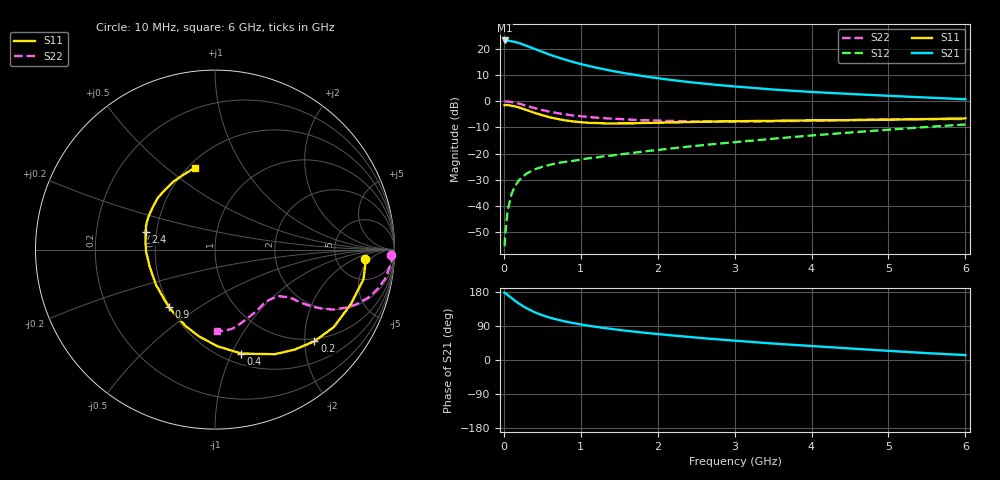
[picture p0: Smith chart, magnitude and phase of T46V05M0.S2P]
! Infineon Technologies  Discrete & RF Semiconductors
! BFR182T
! Si NPN RF Bipolar Junction Transistor in SC75
! VCE = 6 V  IC = 5 mA
! Common Emitter S-Parameters:  October  1999
# GHz  S  MA  R  50
!  f  S11  S21  S12  S22
! GHz  MAG  ANG  MAG  ANG  MAG  ANG  MAG  ANG
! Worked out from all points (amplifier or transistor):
!   36 points, 10 MHz to 6 GHz, reference 50 ohm
!   highest |S21| = 23.2 dB at 10 MHz (marker M1)
!   |S21| within 3 dB of that: start of sweep to 379.6 MHz
!   unconditionally stable (mu >= 1): 1.456 GHz to 4.098 GHz
!   at 250 MHz: K = 0.28, MSG = 25.2 dB, |S12| = -28.8 dB
!   at 1.4 GHz: K = 0.99, MSG = 16.2 dB, |S12| = -20.8 dB
!   at 6 GHz: K = 0.85, MSG = 4.8 dB, |S12| = -8.9 dB
!   lowest NFmin = 1.20 dB at 450 MHz
!   S11 on the Smith chart (normalised r, x): 10 MHz: 10, -3; 200 MHz: 0.94, -2.22; 400 MHz: 0.60, -1.09; 900 MHz: 0.49, -0.38; 2.4 GHz: 0.43, +0.10; 6 GHz: 0.54, +0.63
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0.01  0.8373 -3.4  14.43 177.3  0.0017 86.0  0.9823 -1.7
0.02  0.843 -3.3  14.35 176.7  0.0031 94.5  0.993 -2.0
0.05  0.8438 -11.4  14.36 171.4  0.0082 85.7  0.9812 -5.0
0.1  0.8155 -21.9  13.96 163.6  0.0169 80.5  0.9623 -9.7
0.15  0.7903 -33.1  13.47 155.6  0.0246 73.0  0.9286 -14.0
0.2  0.7535 -42.7  12.84 148.4  0.0312 70.1  0.8923 -17.6
0.25  0.7122 -51.5  12.07 142.0  0.0365 64.9  0.8509 -20.7
0.3  0.671 -60.3  11.32 136.1  0.0419 63.1  0.8119 -23.3
0.4  0.5976 -75.8  9.953 126.0  0.0498 57.6  0.7356 -27.0
0.5  0.5384 -88.6  8.725 118.2  0.0559 54.8  0.6767 -29.0
0.6  0.4915 -100.5  7.694 111.6  0.0609 53.6  0.6274 -30.4
0.7  0.4574 -110.7  6.871 106.3  0.0657 52.7  0.5886 -31.2
0.9  0.4102 -128.7  5.603 97.5  0.0723 52.8  0.5332 -32.1
1.1  0.3854 -143.1  4.721 90.4  0.0811 53.7  0.499 -32.9
1.3  0.3767 -155.3  4.077 84.6  0.0885 54.8  0.4732 -33.8
1.6  0.3766 -169.9  3.365 77.0  0.0999 56.4  0.4469 -35.6
2.2  0.3925 171.2  2.515 64.6  0.1262 59.4  0.4185 -41.0
2.4  0.3989 166.0  2.321 61.0  0.1354 60.0  0.4114 -43.2
3.5  0.4209 145.0  1.669 43.4  0.1917 60.8  0.4133 -56.6
4.5  0.434 130.1  1.373 30.4  0.2519 58.4  0.4347 -70.5
5.5  0.4533 112.5  1.172 18.1  0.3214 54.3  0.4554 -83.0
6  0.469 104.0  1.088 13.0  0.3586 51.1  0.4545 -88.3
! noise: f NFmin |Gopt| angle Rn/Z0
0.45  1.2  0.27  37  0.3
0.9  1.3  0.25  75  0.23
1.8  1.9  0.21  145  0.2
